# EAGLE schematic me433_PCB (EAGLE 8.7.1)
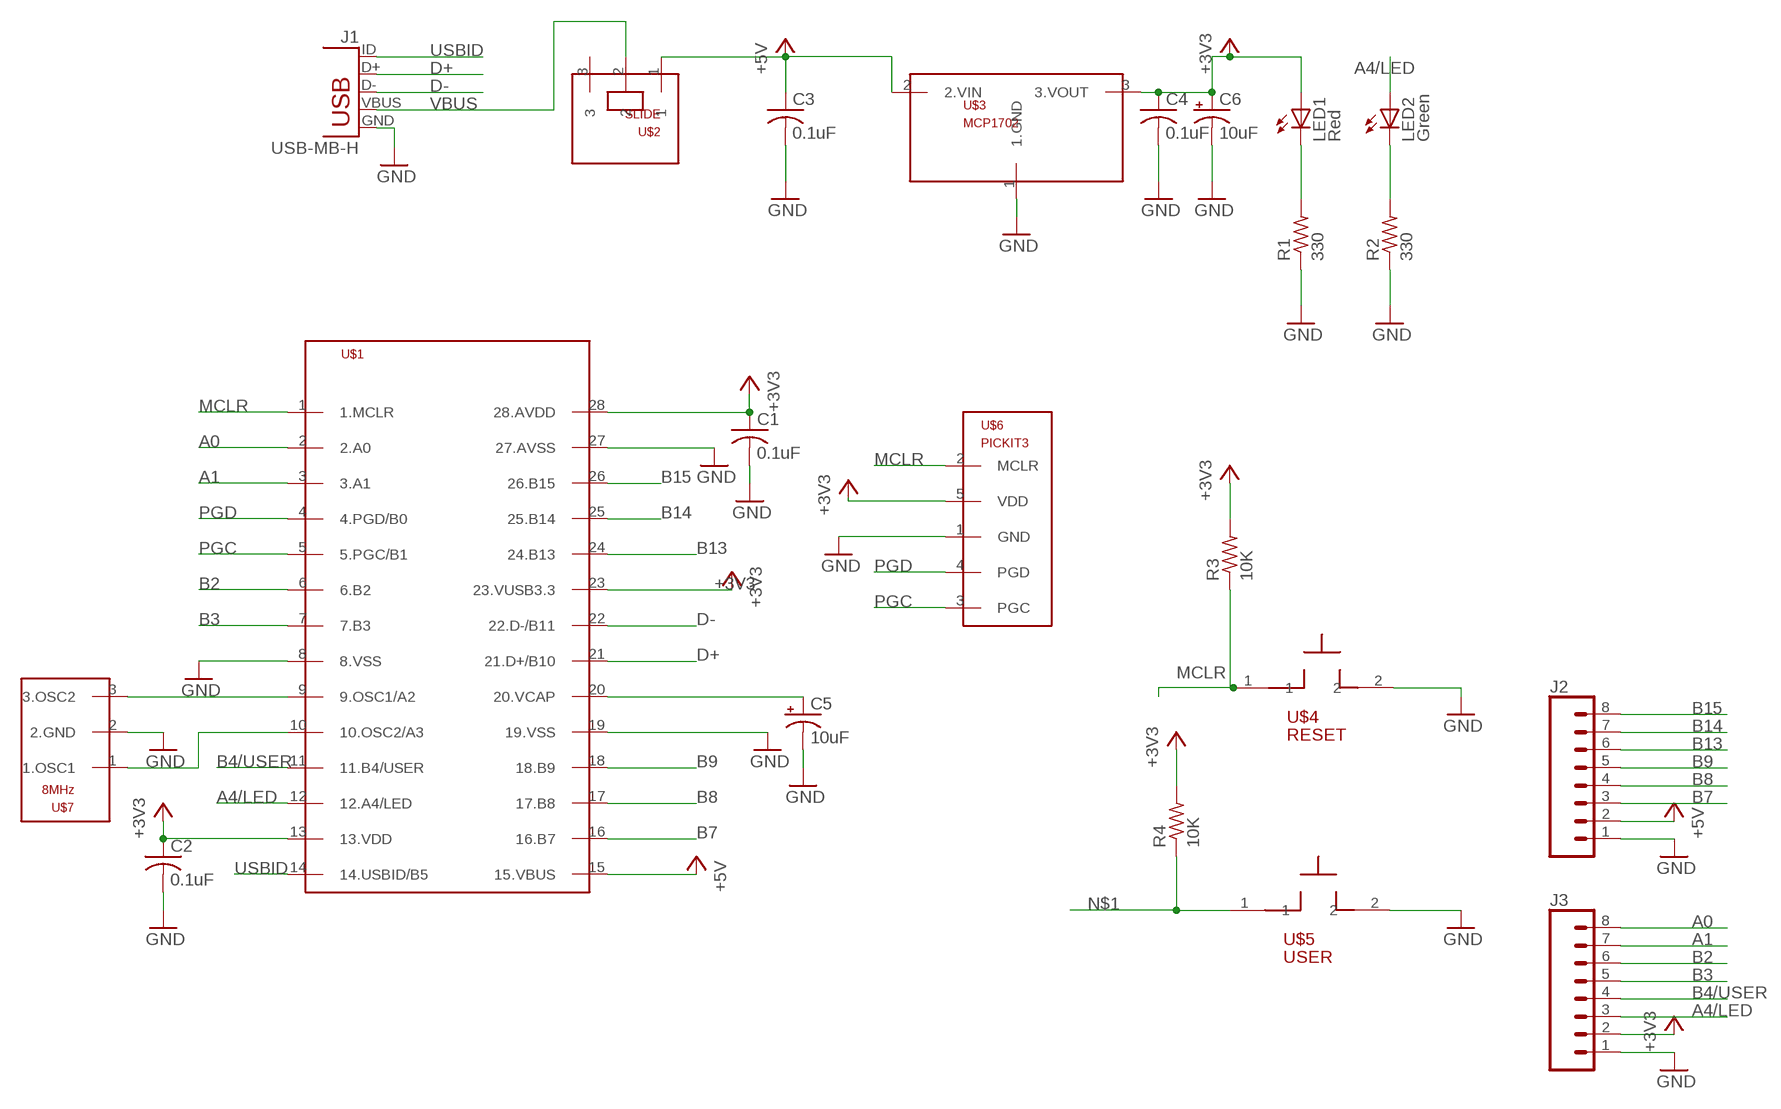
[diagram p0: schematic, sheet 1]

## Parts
C1  0.1uF  C-US025-025X050  [C025-025X050]
C2  0.1uF  C-US025-025X050  [C025-025X050]
C3  0.1uF  C-US025-025X050  [C025-025X050]
C4  0.1uF  C-US025-025X050  [C025-025X050]
C5  10uF  CPOL-USB45181B  [B45181B]
C6  10uF  CPOL-USB45181B  [B45181B]
J1  USB-MB-H  [USB-MB-H]
J2  CONN_08"  [1X08]
J3  CONN_08"  [1X08]
LED1  Red  LED3MM  [LED3MM]
LED2  Green  LED3MM  [LED3MM]
R1  330  R-US_0207/10  [0207/10]
R2  330  R-US_0207/10  [0207/10]
R3  10K  R-US_0207/10  [0207/10]
R4  10K  R-US_0207/10  [0207/10]
U$1  PIC32MX250F138B  [DIL28-3]
U$2  SLIDE  [SLIDE]
U$3  MCP1702  [TO92]
U$4  RESET  PB  [PB]
U$5  USER  PB  [PB]
U$6  PICKIT3  [1X05]
U$7  8MHz  OSC  [OSC]

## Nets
+3V3: C1.1 C2.1 C4.1 C6.+ J3.2 LED1.A R3.2 R4.2 U$1.13(13.VDD) U$1.23(23.VUSB3.3) U$1.28(28.AVDD) U$3.3(3.VOUT) U$6.5(VDD)
+5V: C3.1 J2.2 U$1.15(15.VBUS) U$2.1 U$3.2(2.VIN)
A0: J3.8 U$1.2(2.A0)
A1: J3.7 U$1.3(3.A1)
A4/LED: J3.3 LED2.A U$1.12(12.A4/LED)
B2: J3.6 U$1.6(6.B2)
B3: J3.5 U$1.7(7.B3)
B4/USER: J3.4 U$1.11(11.B4/USER)
B7: J2.3 U$1.16(16.B7)
B8: J2.4 U$1.17(17.B8)
B9: J2.5 U$1.18(18.B9)
B13: J2.6 U$1.24(24.B13)
B14: J2.7 U$1.25(25.B14)
B15: J2.8 U$1.26(26.B15)
D+: J1.D+ U$1.21(21.D+/B10)
D-: J1.D- U$1.22(22.D-/B11)
GND: C1.2 C2.2 C3.2 C4.2 C5.- C6.- J1.GND J2.1 J3.1 R1.1 R2.1 U$1.8(8.VSS) U$1.19(19.VSS) U$1.27(27.AVSS) U$3.1(1.GND) U$4.2 U$5.2 U$6.1(GND) U$7.2(2.GND)
MCLR: R3.1 U$1.1(1.MCLR) U$4.1 U$6.2(MCLR)
N$1: R4.1 U$5.1
N$2: LED1.K(C) R1.2
N$3: LED2.K(C) R2.2
N$4: U$1.10(10.OSC2/A3) U$7.1(1.OSC1)
N$5: U$1.9(9.OSC1/A2) U$7.3(3.OSC2)
N$7: C5.+ U$1.20(20.VCAP)
PGC: U$1.5(5.PGC/B1) U$6.3(PGC)
PGD: U$1.4(4.PGD/B0) U$6.4(PGD)
USBID: J1.ID U$1.14(14.USBID/B5)
VBUS: J1.VBUS U$2.2
Unconnected: U$2.3

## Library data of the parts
C1-C4 = ME433:C-US: CAPACITOR, American symbol
C5 C6 = ME433:CPOL-US: POLARIZED CAPACITOR, American symbol
J1 = ME433:USB: USB Connectors USB-B-PTH is fully proven SKU : PRT-00139/CONN-08278 USB-miniB is fully proven SKU : PRT-00587 USB-A-PCB is untested. USB-A-H is throughly reviewed, but untested. Spark Fun Electronics SKU : PRT-00437 USB-B-SMT is throughly reviewed, but untested. Needs silkscreen touching up.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
J2 J3 = ME433:CONN_08: Multi connection point. Often used as Generic Header-pin footprint for 0.1 inch spaced/style header connections On any of the 0.1 inch spaced packages, you can populate with these: Break Away Headers - Straight (PRT-00116) Break Away Male Headers - Right Angle (PRT-00553) Female Headers (PRT-00115)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; PROD_ID: CONN-08438
LED1 LED2 = led:LED: LED
R1-R4 = ME433:R-US_: RESISTOR, American symbol
U$1 = ME433:PIC32MX250F138B
U$2 = ME433:SLIDE
U$3 = ME433:MCP1702
U$4 U$5 = ME433:PB
U$6 = ME433:PICKIT3
U$7 = ME433:OSC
